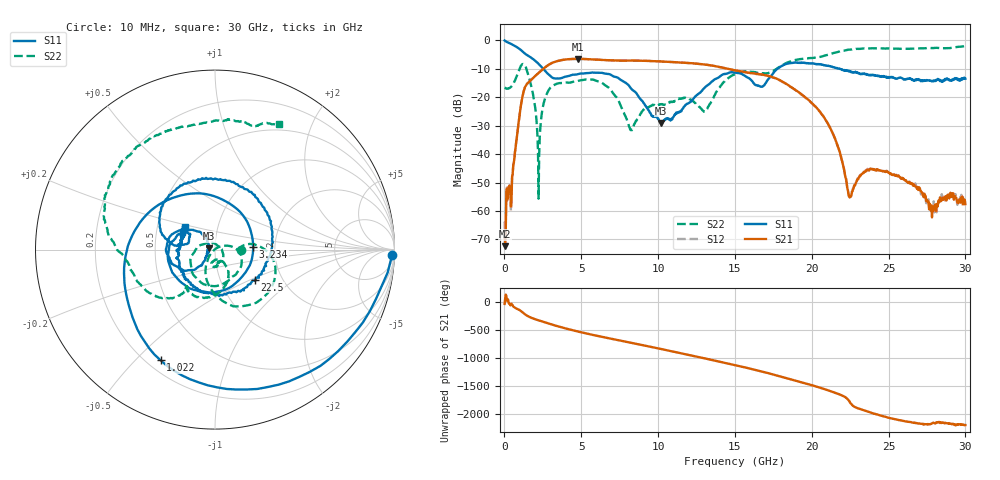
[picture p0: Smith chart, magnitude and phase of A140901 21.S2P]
!  2-Port S-parameters saved by WinCal
! VAR MeasName=S-Parameters (CALIBRATED_DATA) read from VNA (N5244A)
! VAR MeasDate=11/3/2014 9:28:34 AM
! VAR NAME=A140901 21
! VAR FILENAME=A140901 21.S2P
! VAR DATE=11/3/2014 9:28:34 AM
! VAR PHYS_PORTS=1,2
# Hz S RI R 50
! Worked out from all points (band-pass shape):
!   801 points, 10 MHz to 30 GHz, reference 50 ohm
!   highest |S21| = -6.58 dB at 4.771 GHz (marker M1); lowest = -72.4 dB at 47.49 MHz (marker M2)
!   |S21| within 3 dB of the highest: 2.636 GHz to 14.12 GHz (11.48 GHz wide, 137 % of centre)
!   lowest |S11| = -29.1 dB at 10.17 GHz (marker M3), VSWR 1.07, Z = 46.6 + j0.584 ohm
!   |S11| at or under -10 dB: 2.518 GHz to 17.77 GHz (15.25 GHz wide, 150 % of centre); 21.76 GHz to end of sweep
!   |S22| runs from -55.7 to -2.1 dB; largest |S21 - S12| = 0.0049
!   S11 on the Smith chart (normalised r, x): 10 MHz: 23, -55; 1.022 GHz: 0.25, -0.59; 3.234 GHz: 1.54, +0.05; 22.5 GHz: 1.46, -0.53; 30 GHz: 0.69, +0.18
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1e7  0.9866 -0.0309  0.000277 -0.000246  0.000293 -0.000578  0.1465 -0.00107
4.74875e7  0.962 -0.1281  0.000142 0.000195  -0.000265 0.0002  0.145 -0.00317
5.34825e8  0.3537 -0.7528  0.00202 -0.00399  0.00189 -0.00403  0.1635 0.0258
1.022162e9  -0.3031 -0.6166  -0.0534 -0.0214  -0.0535 -0.0214  0.3263 -0.0619
1.696938e9  -0.499 -0.0391  0.0399 0.1928  0.0402 0.1927  -0.0466 -0.1698
2.221762e9  -0.2643 0.2761  0.2368 0.1197  0.2364 0.1196  -0.00149 0.000695
3.233925e9  0.2126 0.0147  0.2082 -0.3552  0.2088 -0.3547  0.1488 -0.0656
4.770912e9  -0.1174 -0.2239  -0.4633 -0.0728  -0.4638 -0.0726  0.0598 -0.1816
5.033325e9  -0.1574 -0.2059  -0.4633 0.0648  -0.4629 0.0655  0.0331 -0.1967
6.382875e9  -0.2633 -0.0365  -0.0104 0.4488  -0.0105 0.4485  -0.1291 -0.1184
7.882375e9  -0.141 0.1104  0.4318 0.0628  0.4313 0.0634  -0.0246 0.0387
1.001916e10  -0.0399 0.0114  -0.1608 -0.3934  -0.1609 -0.3923  0.0194 -0.0692
1.016911e10  -0.0347 0.00625  -0.2163 -0.3626  -0.2159 -0.3615  0.0212 -0.072
1.26058e10  -0.0736 -0.0863  -0.0473 0.3802  -0.0465 0.3807  -0.0155 -0.0693
1.5005e10  -0.2671 0.0307  0.1916 -0.225  0.1874 -0.2256  0.000117 -0.2541
1.684189e10  -0.1532 0.034  -0.2414 -0.0498  -0.2385 -0.0493  -0.1588 -0.2086
2.002832e10  0.0829 0.383  0.0518 -0.0574  0.0524 -0.0566  -0.4765 -0.091
2.145285e10  0.3199 0.0952  -0.0204 -0.00194  -0.0203 -0.00244  -0.5927 0.0778
2.25025e10  0.2234 -0.1666  0.00181 8.04e-06  0.00184 9.5e-06  -0.6092 0.3063
2.501416e10  -0.1834 -0.1163  -0.000406 0.00472  -0.000387 0.0048  -0.262 0.6649
2.778824e10  -0.184 0.0607  0.00122 -0.000255  0.00111 4.32e-05  0.1068 0.72
3e10  -0.1674 0.1271  0.0011 -0.000718  0.00114 -0.000716  0.3588 0.6974
